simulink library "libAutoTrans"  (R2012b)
settings: Solver=ode45  StartTime=0.0  StopTime=10.0  RelTol=1e-3
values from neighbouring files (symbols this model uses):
  ButterflyValvePosition = [0 25 35 50 90 100]    [initAutoTrans.m]
  DownThresholdSpeed = [0 5 20 35; 0 5 20 35; 0 5 25 40; 0 5 30 50; 0 30 50 80; 0 30 50 80]    [initAutoTrans.m]
  DR = 4    [initAutoTrans.m]
  GearNumber = [1 2 3 4]    [initAutoTrans.m]
  GearShiftNumber = [1 2 3 4]    [initAutoTrans.m]
  ThrottleOpenPosition = [0 25 35 50 90 100]    [initAutoTrans.m]
  UpThresholdSpeed = [10 30 50 1000000000000 ; 10 30 50 1000000000000 ; 15 30 50 1000000000000 ; 23 41 60 1000000000000 ; 40 70 100 1000000000000 ; 40 70 100 1000000000000]    [initAutoTrans.m]
undefined symbols (not defined in the file or in its folder): Gear

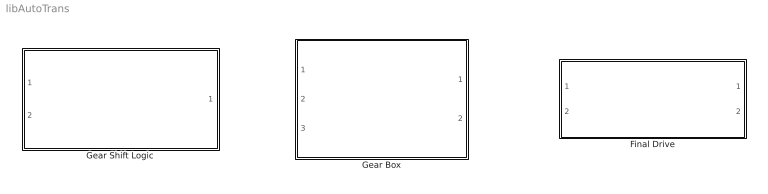
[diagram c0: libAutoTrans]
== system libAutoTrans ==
  Final Drive : Subsystem
  Gear Box : Subsystem
  Gear Shift Logic : Subsystem

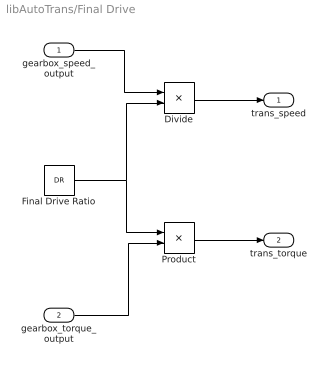
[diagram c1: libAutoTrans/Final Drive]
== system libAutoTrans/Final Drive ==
  gearbox_speed_output : Inport
  gearbox_torque_output : Inport  Port=2
  Divide : Product  Inputs=*/
  Final Drive Ratio : Constant  Value=DR
  Product : Product
  trans_speed : Outport
  trans_torque : Outport  Port=2
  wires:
  Final Drive Ratio/1 -> Divide/2, Product/1
  gearbox_torque_output/1 -> Product/2
  gearbox_speed_output/1 -> Divide/1
  Divide/1 -> trans_speed/1
  Product/1 -> trans_torque/1

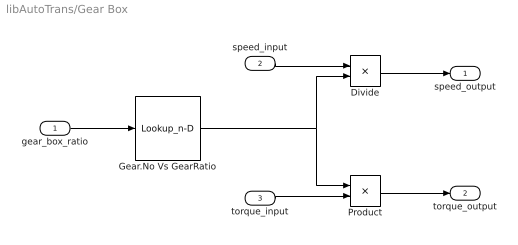
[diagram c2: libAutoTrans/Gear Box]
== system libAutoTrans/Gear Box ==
  gear_box_ratio : Inport
  speed_input : Inport  Port=2
  torque_input : Inport  Port=3
  Divide : Product  Inputs=*/
  Gear.No Vs GearRatio : Lookup_n-D  NumberOfTableDimensions=1  BreakpointsForDimension1=Gear.GearNumber  Table=Gear.GearRatio  RndMeth=Simplest
  Product : Product
  speed_output : Outport
  torque_output : Outport  Port=2
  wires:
  torque_input/1 -> Product/2
  speed_input/1 -> Divide/1
  Divide/1 -> speed_output/1
  Product/1 -> torque_output/1
  gear_box_ratio/1 -> Gear.No Vs GearRatio/1
  Gear.No Vs GearRatio/1 -> Product/1, Divide/2

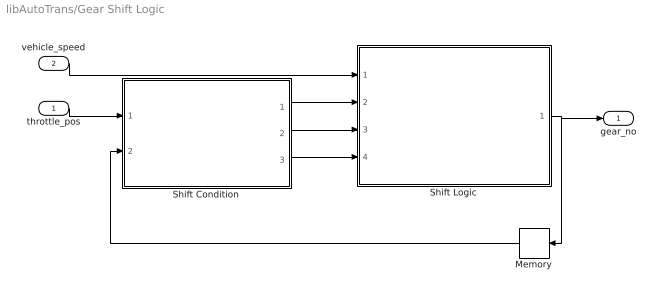
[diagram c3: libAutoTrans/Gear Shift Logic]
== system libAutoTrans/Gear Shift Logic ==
  throttle_pos : Inport
  vehicle_speed : Inport  Port=2
  Memory : Memory  X0=1
  Shift Condition : Subsystem
  Shift Logic : Subsystem
  gear_no : Outport
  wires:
  Shift Condition/1(upper_threshold) -> Shift Logic/2(upper_threshold-speed)
  Shift Condition/2(lower_threshold) -> Shift Logic/3(lower_threshold_speed)
  Shift Condition/3(gear_number) -> Shift Logic/4(gear_no)
  vehicle_speed/1 -> Shift Logic/1(vehicle_ speed)
  throttle_pos/1 -> Shift Condition/1(throttle_pos)
  Shift Logic/1(gear_number) -> Memory/1, gear_no/1
  Memory/1 -> Shift Condition/2(gear_no)

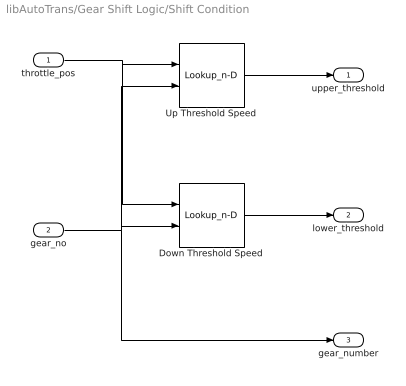
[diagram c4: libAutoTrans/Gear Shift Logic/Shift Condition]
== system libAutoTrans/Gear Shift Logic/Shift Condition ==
  throttle_pos : Inport
  gear_no : Inport  Port=2
  Down Threshold Speed : Lookup_n-D  BreakpointsForDimension1=ThrottleOpenPosition  BreakpointsForDimension2=GearShiftNumber  Table=DownThresholdSpeed  RndMeth=Simplest
  Up Threshold Speed : Lookup_n-D  BreakpointsForDimension1=ButterflyValvePosition  BreakpointsForDimension2=GearNumber  Table=UpThresholdSpeed  RndMeth=Simplest
  upper_threshold : Outport
  lower_threshold : Outport  Port=2
  gear_number : Outport  Port=3
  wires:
  throttle_pos/1 -> Down Threshold Speed/1, Up Threshold Speed/1
  gear_no/1 -> Up Threshold Speed/2, Down Threshold Speed/2, gear_number/1
  Down Threshold Speed/1 -> lower_threshold/1
  Up Threshold Speed/1 -> upper_threshold/1

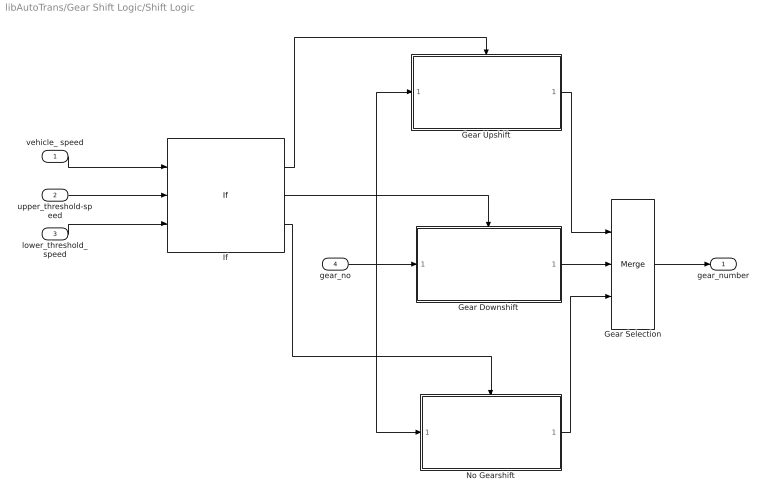
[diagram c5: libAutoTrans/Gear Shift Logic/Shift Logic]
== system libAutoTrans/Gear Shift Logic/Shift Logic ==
  vehicle_ speed : Inport
  upper_threshold-speed : Inport  Port=2
  lower_threshold_speed : Inport  Port=3
  gear_no : Inport  Port=4
  Gear Downshift : Subsystem  TreatAsAtomicUnit=on
  Gear Selection : Merge  Inputs=3
  Gear Upshift : Subsystem  TreatAsAtomicUnit=on
  If : If  NumInputs=3  IfExpression=u1 > u2  ElseIfExpressions=u1<u3
  No Gearshift : Subsystem  TreatAsAtomicUnit=on
  gear_number : Outport
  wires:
  vehicle_ speed/1 -> If/1
  upper_threshold-speed/1 -> If/2
  lower_threshold_speed/1 -> If/3
  If/2 -> Gear Downshift/Action
  If/1 -> Gear Upshift/Action
  If/3 -> No Gearshift/Action
  Gear Selection/1 -> gear_number/1
  gear_no/1 -> Gear Upshift/1(gear_num), No Gearshift/1(gear_number), Gear Downshift/1(gear_number)
  Gear Upshift/1(upshifted_gear_num) -> Gear Selection/1
  Gear Downshift/1(downshifted_gear_no) -> Gear Selection/2
  No Gearshift/1(no_shift) -> Gear Selection/3

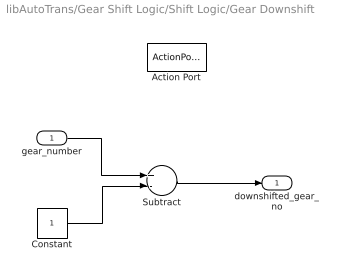
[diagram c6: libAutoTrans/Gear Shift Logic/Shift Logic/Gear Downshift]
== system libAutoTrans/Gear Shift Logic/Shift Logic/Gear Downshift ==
  gear_number : Inport
  Action Port : ActionPort
  Constant : Constant
  Subtract : Sum  Inputs=+-
  downshifted_gear_no : Outport
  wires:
  gear_number/1 -> Subtract/1
  Constant/1 -> Subtract/2
  Subtract/1 -> downshifted_gear_no/1

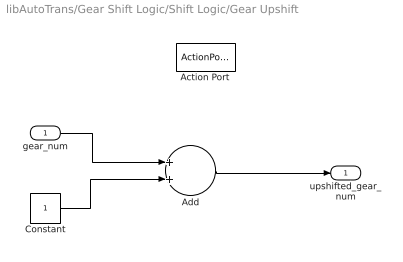
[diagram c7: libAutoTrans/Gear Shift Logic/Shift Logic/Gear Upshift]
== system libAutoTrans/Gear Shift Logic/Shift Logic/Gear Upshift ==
  gear_num : Inport
  Action Port : ActionPort
  Add : Sum
  Constant : Constant
  upshifted_gear_num : Outport
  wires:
  gear_num/1 -> Add/1
  Constant/1 -> Add/2
  Add/1 -> upshifted_gear_num/1

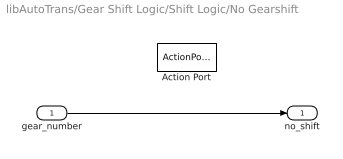
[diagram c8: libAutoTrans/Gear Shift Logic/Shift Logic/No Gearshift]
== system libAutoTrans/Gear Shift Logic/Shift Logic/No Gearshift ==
  gear_number : Inport
  Action Port : ActionPort
  no_shift : Outport
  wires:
  gear_number/1 -> no_shift/1
